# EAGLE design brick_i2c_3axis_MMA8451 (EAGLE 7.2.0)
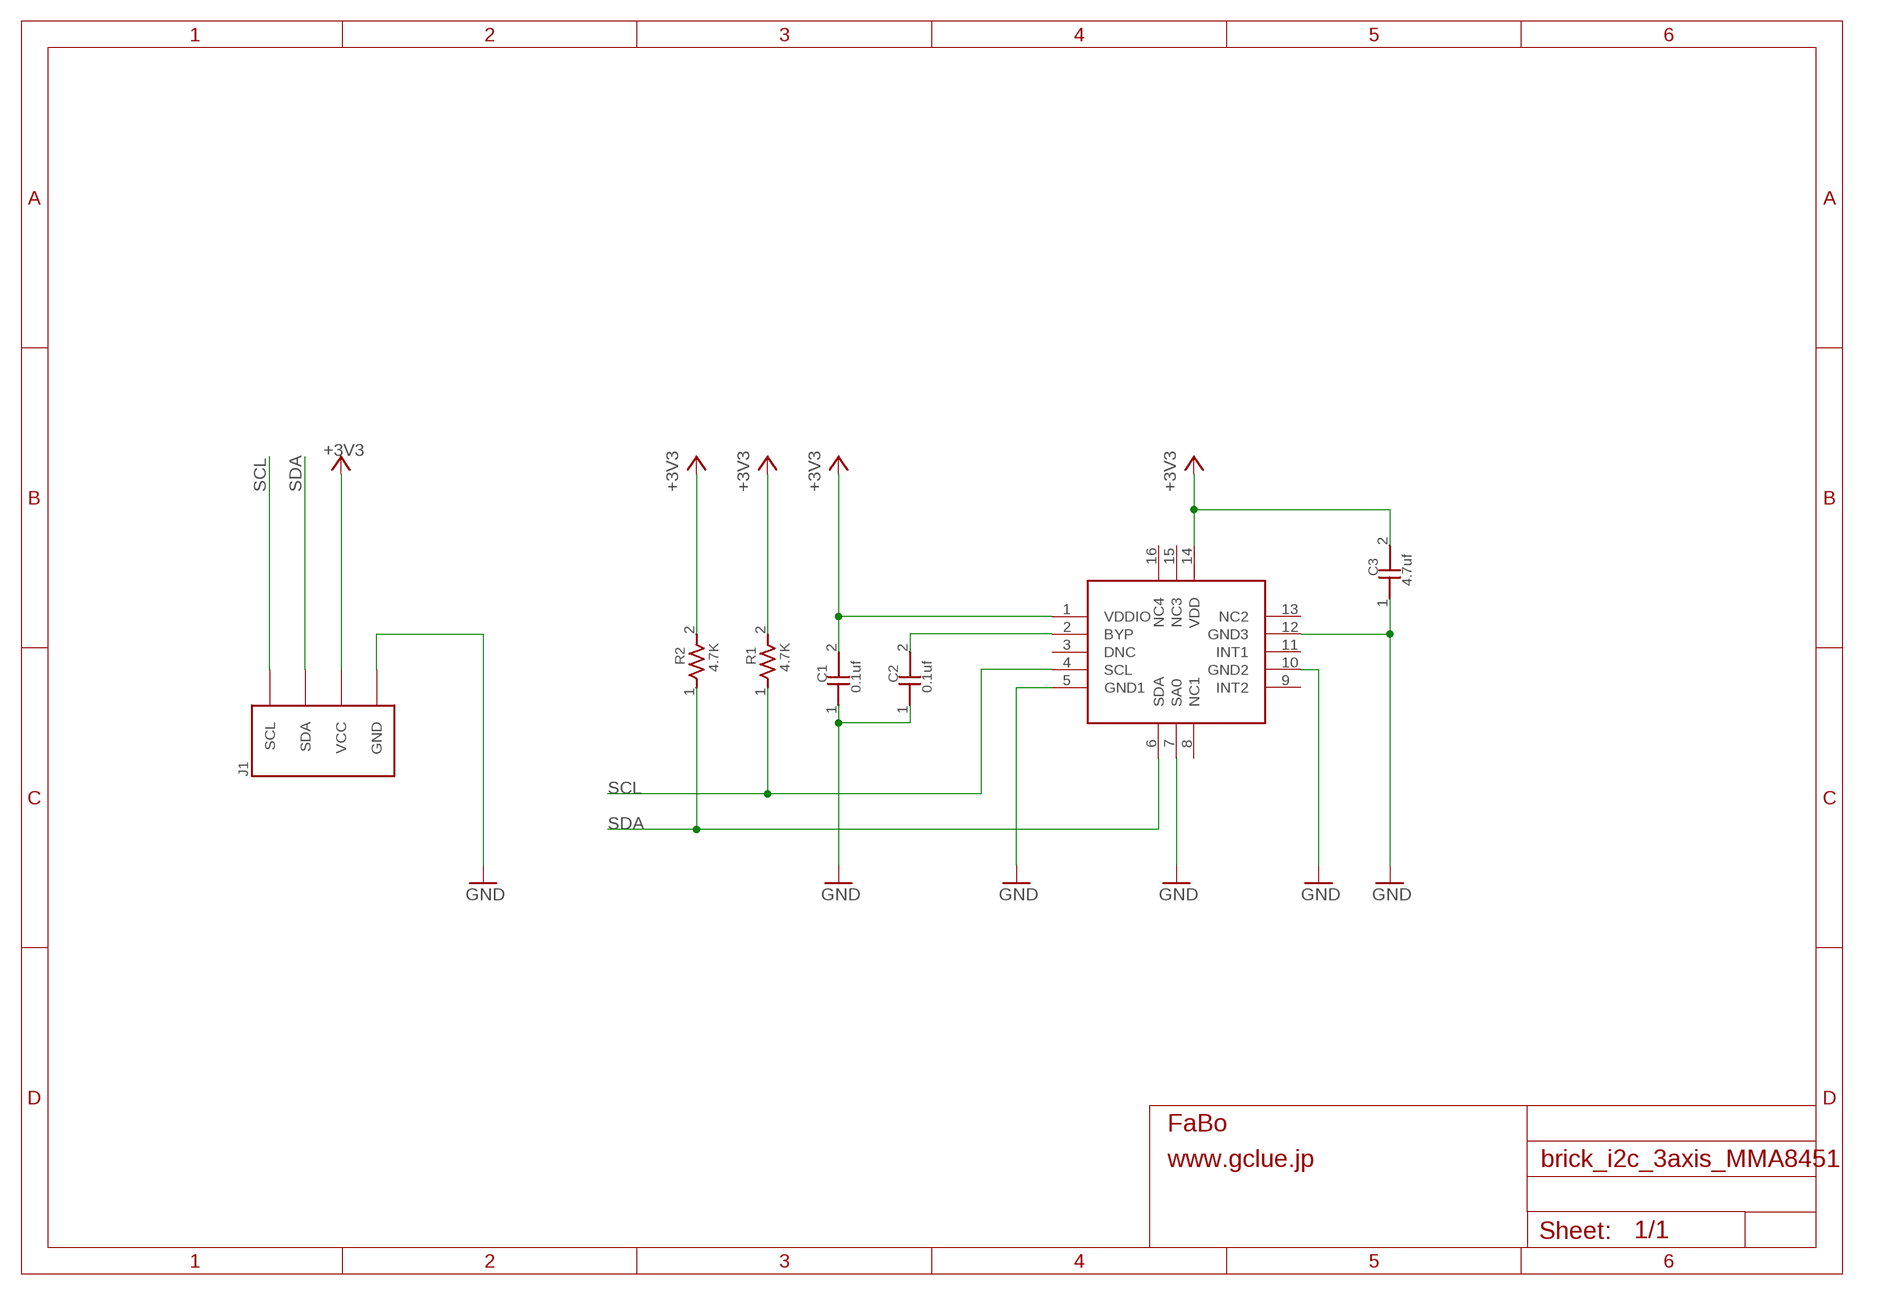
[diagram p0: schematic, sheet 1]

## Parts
C1  0.1uf  CAPACITOR0603  [0603]
C2  0.1uf  CAPACITOR0603  [0603]
C3  4.7uf  CAPACITOR0603  [0603]
J1  BRICK_I2C  [BRICK_I2C]
MMA1  FREESCALE-MMA8451Q  [FREESCALE-MMA8451Q]
R1  4.7K  RESISTOR0603  [0603]
R2  4.7K  RESISTOR0603  [0603]

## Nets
+3V3: C1.2 C3.2 J1.VCC MMA1.1(VDDIO) MMA1.14(VDD) R1.2 R2.2
GND: C1.1 C2.1 C3.1 J1.GND MMA1.5(GND1) MMA1.7(SA0) MMA1.10(GND2) MMA1.12(GND3)
N$1: C2.2 MMA1.2(BYP)
SCL: J1.SCL MMA1.4(SCL) R1.1
SDA: J1.SDA MMA1.6(SDA) R2.1
Unconnected: MMA1.3(DNC) MMA1.8(NC1) MMA1.9(INT2) MMA1.11(INT1) MMA1.13(NC2) MMA1.15(NC3) MMA1.16(NC4)

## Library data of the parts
C1-C3 = GClue-Capacitor:CAPACITOR
J1 = gclue:BRICK_I2C: FaBo Brick 4pin(I2C)
MMA1 = GClue-Mems:FREESCALE-MMA8451Q
R1 R2 = GClue-Resistors:RESISTOR

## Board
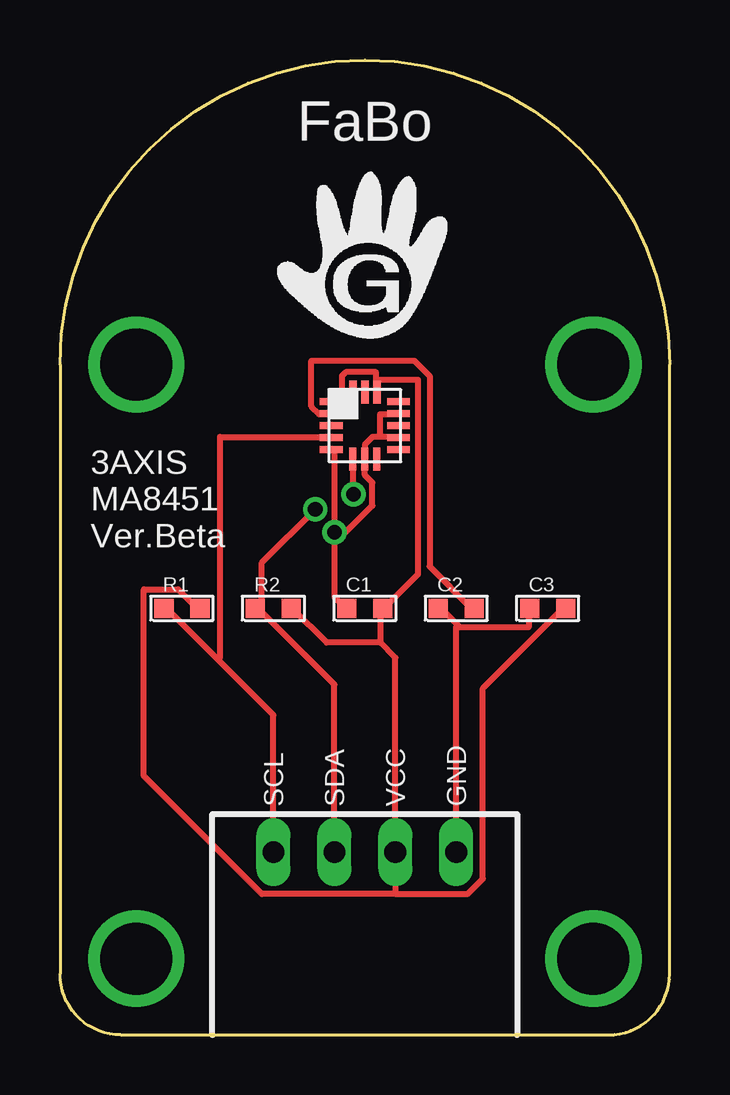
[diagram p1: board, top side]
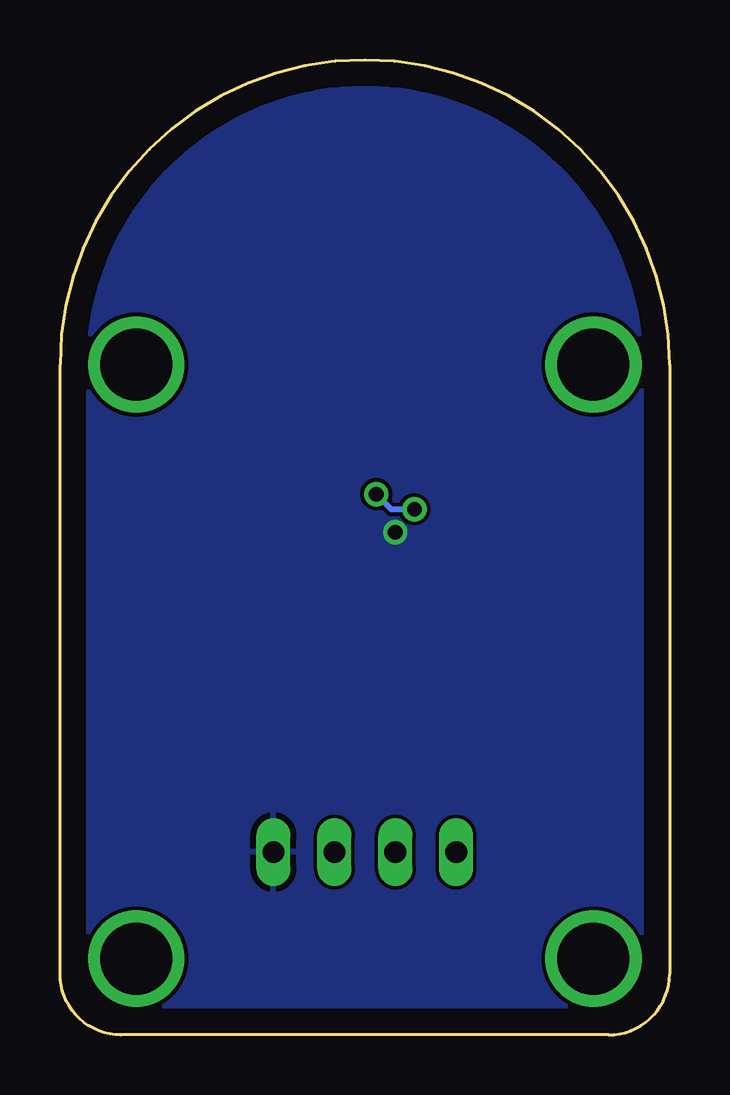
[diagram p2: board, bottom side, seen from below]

Size 25.4 x 40.64 mm. Coordinates in mm from the lower left corner, seen from the top.
Copper layers (1*16): Top 0.035mm / dielectric 1.5mm / Bottom 0.035mm
Design rules "default *": minimum track width 10mil, minimum drill 24mil, track to track 6mil, track to pad 6mil, pad to pad 6mil, via to via 6mil, smd to smd 6mil, copper to edge 40mil, drill to drill 8mil, minimum pad ring 10mil, minimum via ring 8mil, stop-mask expansion 4mil, vias tented up to drill 0mil, thermal gap 10mil

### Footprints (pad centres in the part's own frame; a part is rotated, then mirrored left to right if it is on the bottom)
0603 = smd 0.8 x 0.8: 1 -0.75,0; 2 0.75,0
BRICK_I2C = drill 0.9 long: GND 3.81,-12.7; SCL -3.81,-12.7; SDA -1.27,-12.7; VCC 1.27,-12.7 | drill 3 pad 3.81: P$5 -9.525,7.62; P$6 9.525,7.62; P$7 -9.525,-17.145; P$8 9.525,-17.145
FREESCALE-MMA8451Q = smd 0.95 x 0.305: 1 -1.4,1; 2 -1.4,0.5; 3 -1.4,0; 4 -1.4,-0.5; 5 -1.4,-1; 9 1.4,-1; 10 1.4,-0.5; 11 1.4,0; 12 1.4,0.5; 13 1.4,1 | smd 0.305 x 0.95: 6 -0.5,-1.4; 7 0,-1.4; 8 0.5,-1.4; 14 0.51,1.4; 15 0.01,1.4; 16 -0.49,1.4

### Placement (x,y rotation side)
C1  12.7,17.78 0 top
C2  16.51,17.78 0 top
C3  20.32,17.78 0 top
J1  12.7,20.32 0 top
MMA1  12.7,25.4 0 top
R1  5.08,17.78 0 top
R2  8.89,17.78 0 top

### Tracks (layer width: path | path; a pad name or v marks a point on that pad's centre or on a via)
+3V3
  Top 0.254: 13.18,27.31 13.18,26.83 MMA1.14 | 13.18,27.31 13.18,27.62 11.91,27.62 11.75,27.46 11.75,26.83 11.43,26.51 MMA1.1 | 13.33,16.35 11.11,16.35 9.68,17.78 R2.2 | 13.33,16.35 13.33,17.78 C1.2 13.49,17.78 14.92,19.21 14.92,27.31 13.18,27.31 | 13.97,5.87 8.41,5.87 3.49,10.8 3.49,18.57 4.92,18.57 5.71,17.78 R1.2 | 13.97,5.87 J1.VCC 13.97,15.72 13.33,16.35 | 13.97,5.87 16.99,5.87 17.62,6.51 17.62,14.45 20.95,17.78 C3.2
GND  (via drill 0.61)
  Top 0.254: 13.33,24.92 13.97,24.92 MMA1.10 | 13.33,24.92 13.02,24.92 12.7,24.61 MMA1.7 12.7,23.34 13.02,23.02 13.02,22.07 11.43,20.48 | 13.33,24.92 13.33,25.88 13.97,25.88 MMA1.12 | 11.43,20.48 v11.43,20.96 11.43,24.29 MMA1.5 | 11.43,20.48 11.43,18.26 11.91,17.78 C1.1 | 16.59,17.07 16.67,16.99 19.53,16.99 19.53,17.78 C3.1 | 16.59,17.07 15.88,17.78 C2.1 | J1.GND 16.51,16.99 16.59,17.07
  pour Bottom: -0.64,41.27 26.04,41.27 26.04,-0.63 -0.64,-0.63
N$1
  Top 0.254: C2.2 17.14,17.78 15.4,19.53 15.4,27.46 14.76,28.1 10.48,28.1 10.48,26.19 10.79,25.88 11.27,25.88 MMA1.2
SCL
  Top 0.254: 6.59,15.64 8.89,13.34 J1.SCL | 6.59,15.64 4.44,17.78 R1.1 | MMA1.4 11.27,24.92 6.67,24.92 6.67,15.72 6.59,15.64
SDA  (via drill 0.61)
  Top 0.254: J1.SDA 11.43,14.61 8.25,17.78 R2.1 8.41,17.78 8.41,19.69 v10.64,21.91 | v12.22,22.54 12.22,23.97 MMA1.6
  Bottom 0.254: v12.22,22.54 11.59,21.91 v10.64,21.91

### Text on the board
tPlace: 3AXIS / MA8451 / Ver.Beta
